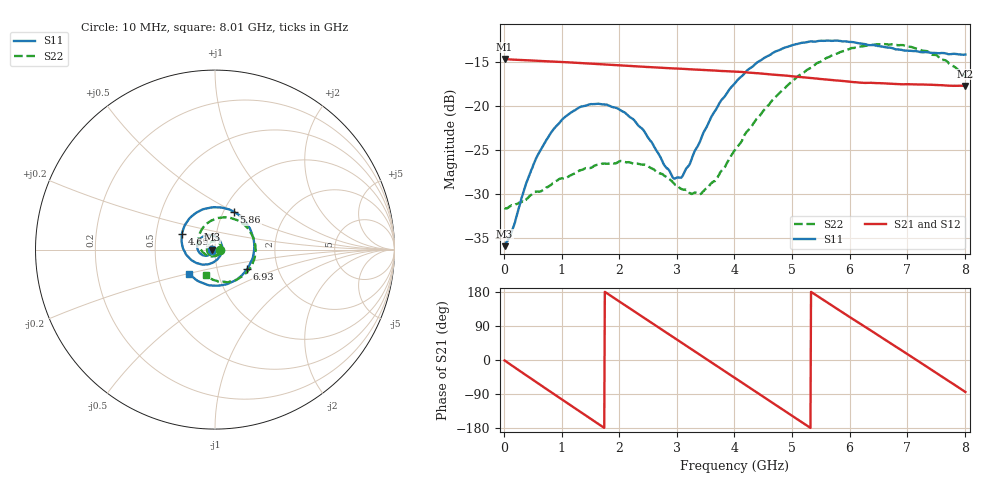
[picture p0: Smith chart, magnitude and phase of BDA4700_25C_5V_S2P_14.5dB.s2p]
!Agilent Technologies,E5071B,MY42404982,A.09.10
!Date: Mon Oct 20 13:33:27 2025
!Data & Calibration Information:
!Freq	S11:SOLT2(ON)	S21:SOLT2(ON)	S12:SOLT2(ON)	S22:SOLT2(ON)
# Hz S RI R 50
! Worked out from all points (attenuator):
!   801 points, 10 MHz to 8.01 GHz, reference 50 ohm
!   highest |S21| = -14.60 dB at 10 MHz (marker M1); lowest = -17.7 dB at 8.01 GHz (marker M2)
!   lowest |S11| = -35.9 dB at 10 MHz (marker M3), VSWR 1.03, Z = 48.4 - j0.124 ohm
!   |S11| at or under -10 dB: start of sweep to end of sweep
!   |S22| runs from -31.6 to -12.9 dB; largest |S21 - S12| = 0.0014
!   S11 on the Smith chart (normalised r, x): 10 MHz: 0.97, -0.00; 4.69 GHz: 0.68, +0.12; 5.86 GHz: 1.12, +0.50; 6.93 GHz: 1.39, -0.32; 8.01 GHz: 0.73, -0.21
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1e7  -0.0159 -0.00128  0.1861 -0.00412  0.1861 -0.00425  0.0263 -0.00102
1.4e8  -0.0172 -0.0095  0.1785 -0.0476  0.1784 -0.0476  0.0264 -0.00712
3.8e8  -0.0261 -0.0249  0.1406 -0.1173  0.1405 -0.1174  0.0209 -0.0206
6.2e8  -0.0436 -0.0341  0.078 -0.164  0.0778 -0.1639  0.01 -0.0311
1.01e9  -0.0809 -0.0233  -0.0451 -0.173  -0.0451 -0.173  -0.0195 -0.0338
1.35e9  -0.0993 0.0106  -0.1338 -0.1147  -0.134 -0.1149  -0.0412 -0.0139
1.71e9  -0.0867 0.0548  -0.1733 -0.0119  -0.1733 -0.0118  -0.0439 0.0172
2.08e9  -0.0448 0.0815  -0.1422 0.0945  -0.1423 0.0945  -0.0232 0.0424
2.42e9  0.00303 0.0732  -0.0633 0.1557  -0.0633 0.1558  0.00746 0.046
2.68e9  0.0299 0.0447  0.0115 0.166  0.0115 0.1661  0.0257 0.0329
2.94e9  0.0387 0.00486  0.0823 0.1424  0.0825 0.1422  0.0343 0.0131
3.08e9  0.035 -0.0179  0.1142 0.1174  0.1135 0.1178  0.0339 -0.000117
3.43e9  -0.00304 -0.0668  0.1587 0.0303  0.1588 0.0304  0.0155 -0.028
4.01e9  -0.1181 -0.0665  0.1067 -0.1163  0.1067 -0.1161  -0.0475 -0.0305
4.69e9  -0.185 0.0853  -0.0666 -0.1359  -0.0663 -0.1363  -0.0915 0.0634
5.35e9  -0.058 0.227  -0.1447 0.00537  -0.1448 0.00508  -0.00514 0.1671
5.86e9  0.1061 0.2094  -0.0847 0.111  -0.0847 0.111  0.1231 0.1643
6.25e9  0.1962 0.1143  0.000979 0.136  0.00242 0.136  0.2015 0.0897
6.68e9  0.2135 -0.0327  0.0915 0.0989  0.0919 0.0987  0.2232 -0.0281
6.93e9  0.1774 -0.1102  0.1231 0.0518  0.1233 0.0513  0.2015 -0.0962
7.47e9  0.0192 -0.2007  0.1141 -0.0675  0.114 -0.0679  0.0776 -0.1805
8.01e9  -0.1428 -0.1362  0.0125 -0.1303  0.0128 -0.1305  -0.0521 -0.1387
